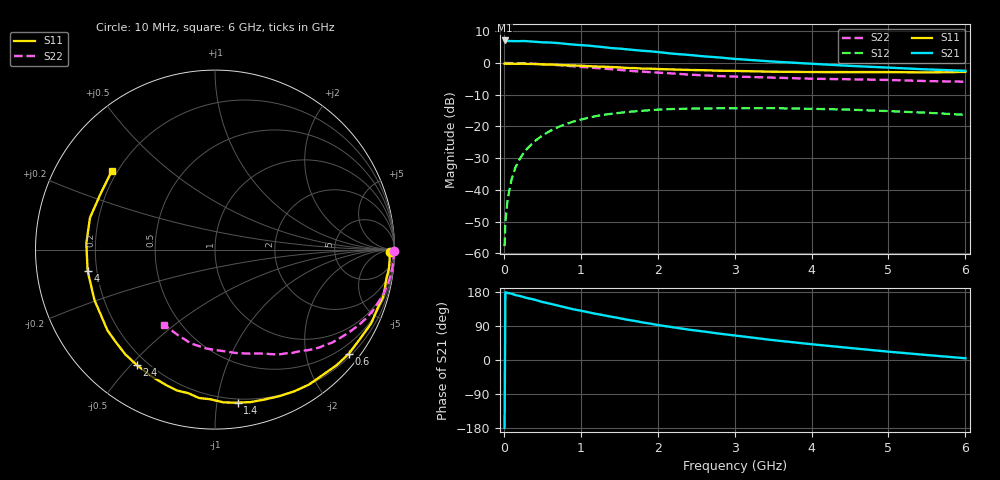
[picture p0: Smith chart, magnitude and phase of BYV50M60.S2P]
! SIEMENS Small Signal Semiconductors
! BFY420
! Si NPN RF SIEGET Grounded Emitter Transistor in MICRO-X
! VCE = 0.5 V  IC = 0.6 mA
! Common Emitter S-Parameters:  October  1996
# GHz  S  MA  R  50
!  f  S11  S21  S12  S22
! GHz  MAG  ANG  MAG  ANG  MAG  ANG  MAG  ANG
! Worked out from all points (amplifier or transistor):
!   36 points, 10 MHz to 6 GHz, reference 50 ohm
!   highest |S21| = 7.1 dB at 10 MHz (marker M1)
!   |S21| within 3 dB of that: start of sweep to 1.69 GHz
!   unconditionally stable (mu >= 1): 4.733 GHz to end of sweep
!   at 250 MHz: K = 0.04, MSG = 17.7 dB, |S12| = -28.6 dB
!   at 1.4 GHz: K = 0.25, MSG = 10.3 dB, |S12| = -16.0 dB
!   at 6 GHz: K = 1.34, MAG = 3.5 dB, |S12| = -16.3 dB
!   S11 on the Smith chart (normalised r, x): 10 MHz: 61, -35; 600 MHz: 0.27, -2.89; 1.4 GHz: 0.17, -1.14; 2.4 GHz: 0.16, -0.52; 4 GHz: 0.16, -0.08; 6 GHz: 0.18, +0.33
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0.01  0.9756 -0.8  2.263 -179.2  0.0013 93.9  0.9994 -0.4
0.02  0.9717 -1.3  2.261 178.8  0.0031 88.3  0.9978 -0.7
0.05  0.9746 -3.3  2.217 176.8  0.0072 85.3  0.9972 -1.8
0.1  0.9749 -6.4  2.215 175.1  0.0146 85.2  0.9946 -3.7
0.15  0.9686 -9.5  2.204 171.3  0.0226 83.0  0.9934 -5.6
0.3  0.9644 -19.0  2.203 163.7  0.0444 77.5  0.9826 -11.0
0.4  0.9624 -25.3  2.158 159.2  0.0585 73.2  0.9721 -14.5
0.5  0.9489 -31.6  2.116 153.0  0.0718 68.9  0.9572 -17.8
0.6  0.9449 -37.9  2.1 148.7  0.0849 64.8  0.9429 -21.2
0.8  0.9206 -49.5  2.003 138.8  0.1081 56.5  0.9059 -27.5
1.1  0.8914 -66.4  1.878 125.9  0.1372 45.9  0.8498 -35.8
1.4  0.862 -81.6  1.713 114.0  0.1583 36.2  0.7969 -43.2
1.6  0.8342 -91.8  1.64 106.4  0.1688 30.5  0.76 -47.6
1.9  0.8132 -105.1  1.53 96.2  0.1805 22.7  0.7179 -53.4
2.2  0.7899 -116.7  1.399 86.3  0.1882 15.7  0.6829 -58.9
2.4  0.7766 -124.2  1.34 80.3  0.1908 11.8  0.6565 -62.4
2.8  0.7553 -137.2  1.221 69.6  0.1935 4.5  0.6218 -68.5
3.5  0.7281 -157.3  1.052 52.4  0.1941 -5.8  0.5873 -78.7
4  0.7195 -170.5  0.973 41.6  0.1896 -12.2  0.5645 -86.7
4.5  0.7178 177.2  0.9 31.7  0.1838 -18.2  0.5536 -94.8
5.5  0.7095 153.8  0.791 13.1  0.1644 -27.4  0.5184 -113.9
6  0.7226 142.8  0.753 4.6  0.1523 -29.7  0.5064 -124.5
